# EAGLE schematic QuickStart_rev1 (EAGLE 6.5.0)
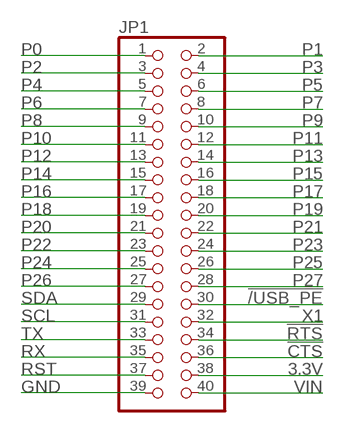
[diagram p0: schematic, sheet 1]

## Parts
JP1  PINHD-2X20  [2X20]

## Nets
3.3V: JP1.38
!/USB_PE: JP1.30
!CTS: JP1.36
!RTS: JP1.34
GND: JP1.39
P0: JP1.1
P1: JP1.2
P2: JP1.3
P3: JP1.4
P4: JP1.5
P5: JP1.6
P6: JP1.7
P7: JP1.8
P8: JP1.9
P9: JP1.10
P10: JP1.11
P11: JP1.12
P12: JP1.13
P13: JP1.14
P14: JP1.15
P15: JP1.16
P16: JP1.17
P17: JP1.18
P18: JP1.19
P19: JP1.20
P20: JP1.21
P21: JP1.22
P22: JP1.23
P23: JP1.24
P24: JP1.25
P25: JP1.26
P26: JP1.27
P27: JP1.28
RST: JP1.37
RX: JP1.35
SCL: JP1.31
SDA: JP1.29
TX: JP1.33
VIN: JP1.40
X1: JP1.32

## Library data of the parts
JP1 = pinhead:PINHD-2X20: PIN HEADER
